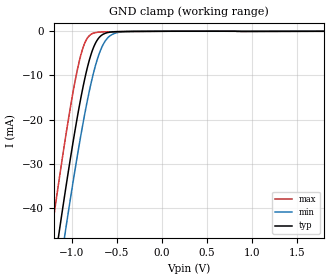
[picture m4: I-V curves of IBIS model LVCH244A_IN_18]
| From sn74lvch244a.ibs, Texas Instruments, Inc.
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[Model]   LVCH244A_IN_18
Model_type  Input
Vinl=0.5775
Vinh=1.2675
| variable   typ   min   max
C_comp   3.40pF   3.13pF   3.94pF
[Temperature Range]   40   100   -40
| Ambient temperature   25   85   -40
[Voltage range]   1.8   1.65   1.95
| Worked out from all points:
|   GND clamp passes 1 mA (typ) near -0.68 V on its own axis
[GND Clamp]
| LVCH244A_IN_18
|   Voltage   I(typ)   I(min)   I(max)
-5.5V     -732.8mA   -739.3mA   -725.1mA
-1.25V    -60.93mA   -70.17mA   -49.08mA
-1.22V    -56.63mA   -65.89mA   -44.74mA
-1.145V   -46.08mA   -55.35mA   -34.15mA
-1.08V    -37.21mA   -46.44mA   -25.35mA
-1.06V    -34.55mA   -43.76mA   -22.74mA
-945mV    -20.16mA   -28.98mA   -9.367mA
-855mV    -10.65mA   -18.58mA   -2.618mA
-735mV    -2.605mA   -7.606mA   -293.4uA
-660mV    -772.5uA   -3.334mA   -154.9uA
-580mV    -217.7uA   -1.101mA   -117.2uA
1.8V      1.115nA    83.1nA     -29.87pA
